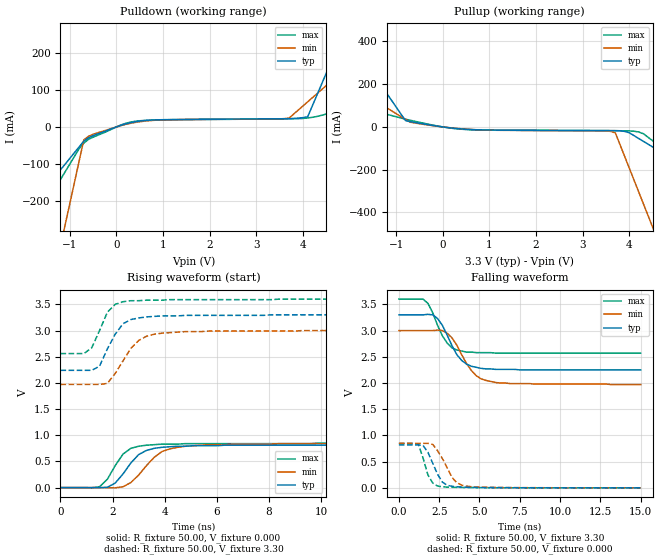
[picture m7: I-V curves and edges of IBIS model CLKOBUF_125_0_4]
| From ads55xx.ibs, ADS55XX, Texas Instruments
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|   Model CLKOBUF_125_0_4
[Model]   CLKOBUF_125_0_4
Model_type   Output
Polarity   Non-Inverting
Vmeas =   1.65V
C_comp   2pf   2pf   2pf
[Temperature Range]   50.00   0.10k   -20.00
[Voltage Range]   3.30V   3.00V   3.60V
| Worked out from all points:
|   slope of the pulldown table from 0 to 0.495 V, typ, clamps not added: 31.6 ohm
|   slope of the pullup table from 0 to 0.495 V, typ, clamps not added: 45.6 ohm
|   rising waveform, R_fixture 50.00, V_fixture 0.000: 20-80 % time 863ps typ, 1ns min, 698ps max; typ from 0 V to 0.82 V
|   rising waveform, R_fixture 50.00, V_fixture 3.30: 20-80 % time 717ps typ, 874ps min, 595ps max; typ from 2.24 V to 3.3 V
|   falling waveform, R_fixture 50.00, V_fixture 3.30: 20-80 % time 1.1ns typ, 1.25ns min, 956ps max; typ from 3.3 V to 2.25 V
|   falling waveform, R_fixture 50.00, V_fixture 0.000: 20-80 % time 756ps typ, 925ps min, 574ps max; typ from 0.82 V to 0.001 V
[Pulldown]
| voltage   I(typ)   I(min)   I(max)
-3.3V     -442.8mA   -1.531A    -582.2mA
-2.3V     -287.3mA   -955.5mA   -372.8mA
-1.9V     -225.1mA   -725.5mA   -289.1mA
-1.5V     -162.9mA   -495.4mA   -205.3mA
-1V       -85.18mA   -207.8mA   -100.6mA
-700mV    -38.53mA   -35.22mA   -43.96mA
200mV     8.22mA     6.96mA     9.79mA
3.7V      22.36mA    23.79mA    22.07mA
4.1V      27.5mA     67.99mA    24.24mA
4.9V      264.3mA    156.4mA    47.82mA
5.9V      560.3mA    266.9mA    80.27mA
6.6V      767.5mA    344.2mA    103mA
[Pullup]
| voltage   I(typ)   I(min)   I(max)
-3.3V     824.9mA    370.6mA    179.3mA
-2.3V     506.8mA    236.6mA    122.1mA
-2.1V     443.2mA    209.7mA    110.7mA
-800mV    29.65mA    35.55mA    36.29mA
-600mV    20.97mA    18.3mA     26.49mA
500mV     -10.93mA   -10.34mA   -12.15mA
3.6V      -17.06mA   -20.85mA   -17.69mA
3.7V      -17.27mA   -28.02mA   -17.77mA
4V        -27.45mA   -193.6mA   -18.62mA
4.2V      -54.03mA   -304mA     -23.54mA
4.5V      -93.9mA    -469.6mA   -64.81mA
6.6V      -373mA     -1.629A    -412.8mA
[Ramp]
| variable   typ   min   max
dV/dt_r   0.49/0.81n   0.51/0.99n   0.51/0.66n
dV/dt_f   0.63/1.10n   0.62/1.22n   0.62/0.93n
R_load = 50.00
[Rising Waveform]
R_fixture = 50.00
V_fixture = 0.000
V_fixture_min = 0.000
V_fixture_max = 0.000
| time   V(typ)   V(min)   V(max)
0s        31.29nV    40.15nV    63.42nV
1.5ns     -2.91mV    38.31uV    15.52mV
1.8ns     6.75mV     -2.04mV    160mV
2.1ns     86.23mV    -5.03mV    420mV
2.4ns     260mV      16.06mV    640mV
3ns       630mV      240mV      790mV
3.3ns     710mV      420mV      810mV
3.9ns     770mV      690mV      830mV
4.8ns     790mV      790mV      840mV
15ns      820mV      840mV      850mV
[Rising Waveform]
R_fixture = 50.00
V_fixture = 3.30
V_fixture_min = 3.00
V_fixture_max = 3.60
| time   V(typ)   V(min)   V(max)
0s        2.24V      1.97V      2.56V
900ps     2.24V      1.97V      2.56V
1.2ns     2.24V      1.97V      2.67V
1.5ns     2.32V      1.97V      3V
1.8ns     2.65V      1.99V      3.35V
2.1ns     2.93V      2.18V      3.5V
2.4ns     3.13V      2.42V      3.55V
3ns       3.24V      2.81V      3.57V
3.9ns     3.28V      2.95V      3.58V
15ns      3.3V       3V         3.6V
[Falling Waveform]
R_fixture = 50.00
V_fixture = 3.30
V_fixture_min = 3.00
V_fixture_max = 3.60
| time   V(typ)   V(min)   V(max)
0s        3.3V       3V         3.6V
1.5ns     3.3V       3V         3.6V
1.8ns     3.31V      3V         3.52V
2.1ns     3.3V       3V         3.34V
2.7ns     3.1V       3V         2.9V
3.6ns     2.54V      2.72V      2.63V
4.2ns     2.36V      2.37V      2.59V
4.8ns     2.3V       2.14V      2.58V
6ns       2.26V      2.01V      2.57V
15ns      2.25V      1.97V      2.57V
[Falling Waveform]
R_fixture = 50.00
V_fixture = 0.000
V_fixture_min = 0.000
V_fixture_max = 0.000
| time   V(typ)   V(min)   V(max)
0s        820mV      850mV      850mV
1.2ns     820mV      850mV      840mV
1.5ns     810mV      850mV      570mV
1.8ns     680mV      850mV      250mV
2.1ns     470mV      830mV      93.28mV
2.4ns     260mV      710mV      36.1mV
2.7ns     110mV      560mV      21.51mV
3.3ns     30.21mV    200mV      12.35mV
4.2ns     12.83mV    33.71mV    7.43mV
15ns      1.24mV     1.56mV     1.29mV
